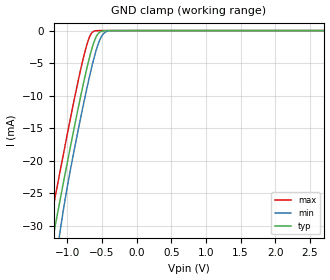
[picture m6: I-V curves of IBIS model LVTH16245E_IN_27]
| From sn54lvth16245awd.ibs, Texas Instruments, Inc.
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[Model]   LVTH16245E_IN_27
Model_type  Input
Vinl=0.945
Vinh=1.75
| variable   typ   min   max
C_comp   2.17pF   1.41pF   2.70pF
[Temperature Range]   40   100   -40
| Ambient temperature   25   85   -40
[Voltage range]   2.7   2.7   2.7
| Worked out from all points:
|   GND clamp passes 1 mA (typ) near -0.59 V on its own axis
[GND Clamp]
| LVTH16245E_IN_27
|   Voltage   I(typ)   I(min)   I(max)
-2.7V     -241.2mA   -262.7mA   -214.2mA
-1.27V    -35.73mA   -45.12mA   -30.82mA
-1.18V    -30.22mA   -36.75mA   -25.77mA
-1.105V   -26mA      -30.83mA   -21.6mA
-975mV    -18.86mA   -22.45mA   -14.51mA
-775mV    -8.44mA    -11.68mA   -4.447mA
-685mV    -4.298mA   -7.265mA   -1.099mA
-615mV    -1.738mA   -4.194mA   -91.47uA
-560mV    -525uA     -2.205mA   -6.893uA
-505mV    -96.03uA   -845.6uA   -485.1nA
-365mV    -669.1nA   -19.3uA    -560pA
2.7V      9.886pA    968.6pA    8.595pA
